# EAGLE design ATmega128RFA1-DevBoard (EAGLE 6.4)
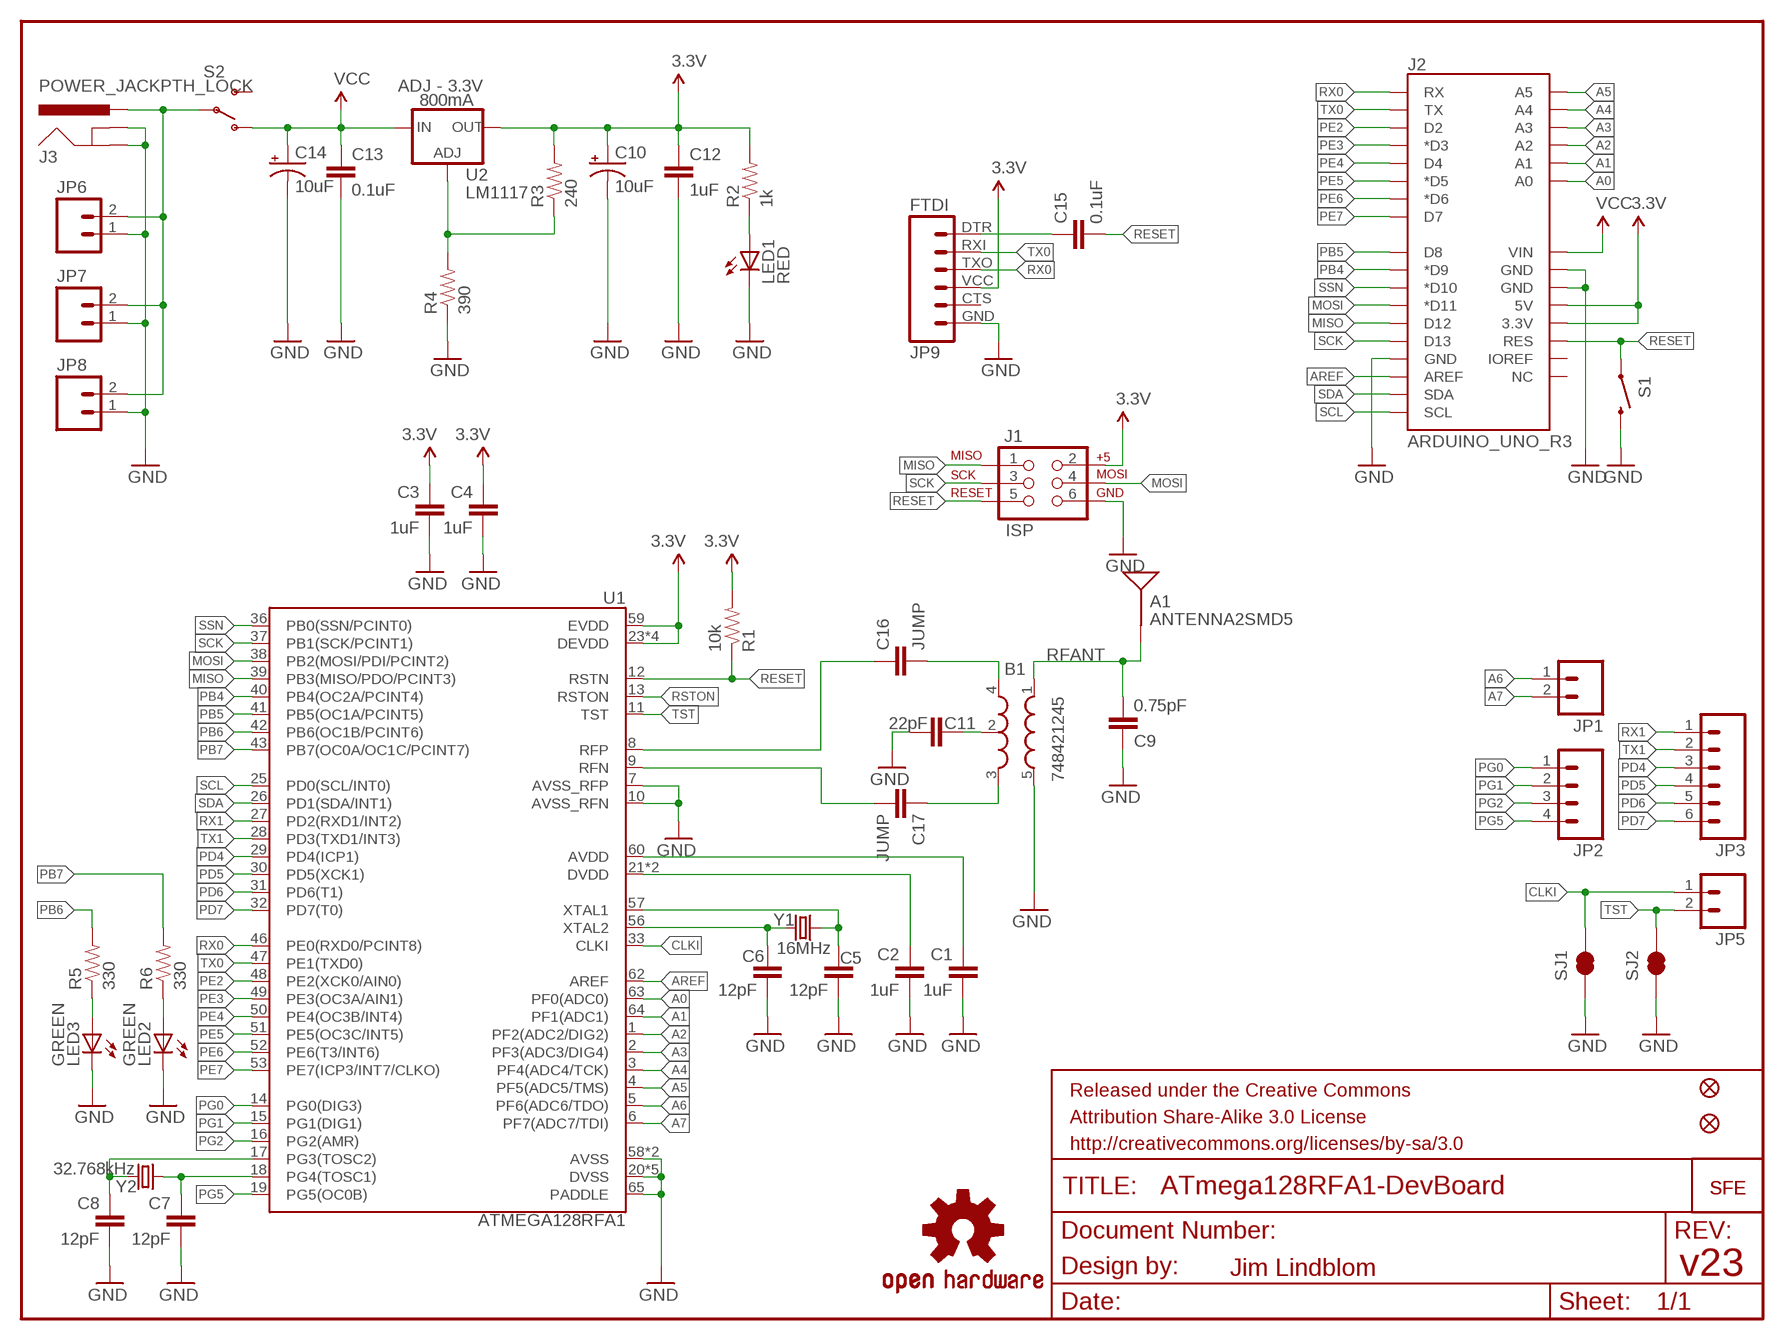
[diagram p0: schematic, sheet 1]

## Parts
A1  ANTENNA2SMD5  [ANTENNA-CHIP5]
B1  748421245  BALUN0805  [BALUN]
C1  1uF  CAP0402-CAP  [0402-CAP]
C2  1uF  CAP0402-CAP  [0402-CAP]
C3  1uF  CAP0402-CAP  [0402-CAP]
C4  1uF  CAP0402-CAP  [0402-CAP]
C5  12pF  CAP0402-CAP  [0402-CAP]
C6  12pF  CAP0402-CAP  [0402-CAP]
C7  12pF  CAP0402-CAP  [0402-CAP]
C8  12pF  CAP0402-CAP  [0402-CAP]
C9  0.75pF  CAP0402-CAP  [0402-CAP]
C10  10uF  CAP_POL1206  [EIA3216]
C11  22pF  CAP0402-CAP  [0402-CAP]
C12  1uF  CAP0402-CAP  [0402-CAP]
C13  0.1uF  CAP0402-CAP  [0402-CAP]
C14  10uF  CAP_POL1206  [EIA3216]
C15  0.1uF  CAP0402-CAP  [0402-CAP]
C16  JUMP  CAP0402-CAP  [0402-CAP]
C17  JUMP  CAP0402-CAP  [0402-CAP]
FID1  FIDUCIALUFIDUCIAL  [MICRO-FIDUCIAL]
FID2  FIDUCIALUFIDUCIAL  [MICRO-FIDUCIAL]
J1  ISP  AVR_SPI_PRG_6NS  [2X3-NS]
J2  ARDUINO_UNO_R3  [ARDUINO_UNO_R3]
J3  POWER_JACKPTH_LOCK  [POWER_JACK_PTH_LOCK]
JP1  M021X02_NO_SILK  [1X02_NO_SILK]
JP2  M041X04_NO_SILK  [1X04_NO_SILK]
JP3  M06SIP-NS  [1X06_NS]
JP4  LOGO-SFENEW  [SFE-NEW-WEBLOGO]
JP5  M021X02_NO_SILK  [1X02_NO_SILK]
JP6  M02JST-PTH-2  [JST-2-PTH]
JP7  M021X02_NO_SILK  [1X02_NO_SILK]
JP8  M023.5MM-NO_SILK  [SCREWTERMINAL-3.5MM-2-NS]
JP9  FTDI  FTDI_BASICPTH  [FTDI_BASIC]
JP10  LOGO-SFENEW  [SFE-NEW-WEBLOGO]
LED1  RED  LED0603  [LED-0603]
LED2  GREEN  LED0603  [LED-0603]
LED3  GREEN  LED0603  [LED-0603]
R1  10k  RESISTOR0402-RES  [0402-RES]
R2  1k  RESISTOR0402-RES  [0402-RES]
R3  240  RESISTOR0402-RES  [0402-RES]
R4  390  RESISTOR0402-RES  [0402-RES]
R5  330  RESISTOR0402-RES  [0402-RES]
R6  330  RESISTOR0402-RES  [0402-RES]
S1  SWITCH-MOMENTARY-2SMD  [TACTILE_SWITCH_SMD]
S2  SWITCH-SPST-SMD-A  [SWITCH-SPST-SMD-A]
SJ1  SOLDERJUMPERTRACE  [SJ_2S-TRACE]
SJ2  SOLDERJUMPERTRACE  [SJ_2S-TRACE]
U1  ATMEGA128RFA1  [QFN-64]
U2  LM1117  V_REG_317SMD  [SOT223]
U$1  OSHW-LOGOS  [OSHW-LOGO-S]
Y1  16MHz  CRYSTAL5X3  [CRYSTAL-SMD-5X3]
Y2  32.768kHz  CRYSTAL32-SMD  [CRYSTAL-32KHZ-SMD]

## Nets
3.3V: C3.1 C4.1 C10.A(+) C12.1 J1.2 J2.3.3V J2.5V JP9.VCC R1.2 R2.2 R3.2 U1.23(DEVDD) U1.34(DEVDD) U1.44(DEVDD) U1.54(DEVDD) U1.59(EVDD) U2.2(OUT)
A0: J2.A0 U1.63(PF0(ADC0))
A1: J2.A1 U1.64(PF1(ADC1))
A2: J2.A2 U1.1(PF2(ADC2/DIG2))
A3: J2.A3 U1.2(PF3(ADC3/DIG4))
A4: J2.A4 U1.3(PF4(ADC4/TCK))
A5: J2.A5 U1.4(PF5(ADC5/TMS))
A6: JP1.1 U1.5(PF6(ADC6/TDO))
A7: JP1.2 U1.6(PF7(ADC7/TDI))
AREF: J2.AREF U1.62(AREF)
AVDD: C1.1 U1.60(AVDD)
CLKI: JP5.1 SJ1.2 U1.33(CLKI)
DTR: C15.1 JP9.DTR
DVDD: C2.1 U1.21(DVDD) U1.22(DVDD)
FB: R3.1 R4.2 U2.1(ADJ)
GND: B1.5(GND) C1.2 C2.2 C3.2 C4.2 C5.2 C6.2 C7.2 C8.2 C9.1 C10.C(-) C11.2 C12.2 C13.2 C14.C(-) J1.6 J2.GND@0(GND) J2.GND@1(GND) J2.GND@2(GND) J3.GND J3.GNDBREAK JP6.1 JP7.1 JP8.1 JP9.GND LED1.C LED2.C LED3.C R4.1 S1.3 SJ1.1 SJ2.1 U1.7(AVSS_RFP) U1.10(AVSS_RFN) U1.20(DVSS) U1.24(DVSS) U1.35(DVSS) U1.45(DVSS) U1.55(DVSS) U1.58(AVSS) U1.61(AVSS) U1.65(PADDLE)
MISO: J1.1 J2.D12 U1.39(PB3(MISO/PDO/PCINT3))
MOSI: J1.4 J2.D11(*D11) U1.38(PB2(MOSI/PDI/PCINT2))
N$2: LED1.A R2.1
N$3: C5.1 U1.57(XTAL1) Y1.3
N$4: C6.1 U1.56(XTAL2) Y1.1
N$5: C7.1 U1.18(PG4(TOSC1)) Y2.X1
N$6: C8.1 U1.17(PG3(TOSC2)) Y2.X2
N$7: B1.2(GND) C11.1
N$8: LED3.A R5.1
N$9: J3.PWR JP6.2 JP7.2 JP8.2 S2.2(P)
N$10: B1.4(OUT1) C16.2
N$11: B1.3(OUT2) C17.1
N$13: LED2.A R6.1
PB4: J2.D9(*D9) U1.40(PB4(OC2A/PCINT4))
PB5: J2.D8 U1.41(PB5(OC1A/PCINT5))
PB6: R5.2 U1.42(PB6(OC1B/PCINT6))
PB7: R6.2 U1.43(PB7(OC0A/OC1C/PCINT7))
PD4: JP3.3 U1.29(PD4(ICP1))
PD5: JP3.4 U1.30(PD5(XCK1))
PD6: JP3.5 U1.31(PD6(T1))
PD7: JP3.6 U1.32(PD7(T0))
PE2: J2.D2 U1.48(PE2(XCK0/AIN0))
PE3: J2.D3(*D3) U1.49(PE3(OC3A/AIN1))
PE4: J2.D4 U1.50(PE4(OC3B/INT4))
PE5: J2.D5(*D5) U1.51(PE5(OC3C/INT5))
PE6: J2.D6(*D6) U1.52(PE6(T3/INT6))
PE7: J2.D7 U1.53(PE7(ICP3/INT7/CLKO))
PG0: JP2.1 U1.14(PG0(DIG3))
PG1: JP2.2 U1.15(PG1(DIG1))
PG2: JP2.3 U1.16(PG2(AMR))
PG5: JP2.4 U1.19(PG5(OC0B))
RESET: C15.2 J1.5 J2.RES R1.1 S1.1 U1.12(RSTN)
RFANT: A1.FEED(SIGNAL) B1.1(IN) C9.2
RFN: C17.2 U1.9(RFN)
RFP: C16.1 U1.8(RFP)
RSTON: U1.13(RSTON)
RX0: J2.RX JP9.TXO U1.46(PE0(RXD0/PCINT8))
RX1: JP3.1 U1.27(PD2(RXD1/INT2))
SCK: J1.3 J2.D13 U1.37(PB1(SCK/PCINT1))
SCL: J2.SCL U1.25(PD0(SCL/INT0))
SDA: J2.SDA U1.26(PD1(SDA/INT1))
SSN: J2.D10(*D10) U1.36(PB0(SSN/PCINT0))
TST: JP5.2 SJ2.2 U1.11(TST)
TX0: J2.TX JP9.RXI U1.47(PE1(TXD0))
TX1: JP3.2 U1.28(PD3(TXD1/INT3))
VCC: C13.1 C14.A(+) J2.VIN S2.1(O) U2.3(IN)
Unconnected: J2.IOREF J2.NC JP9.CTS S2.3(S)

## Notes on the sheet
- ADJ - 3.3V
- 800mA
- Jim Lindblom | v23

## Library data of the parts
A1 = SparkFun-RF:ANTENNA2: Chip antenna
B1 = SparkFun-RF:BALUN: 0805 footprint balun- Ember 351/357
C1-C9 C11-C13 C15 = SparkFun-Passives:CAP: Capacitor
C10 C14 = SparkFun-Passives:CAP_POL: Capacitor Polarized
C16 C17 = SparkFun:CAP: Capacitor
FID1 FID2 = SparkFun-Aesthetics:FIDUCIAL: Fiducial Alignment Points
J1 = SparkFun-Connectors:AVR_SPI_PRG_6: AVR ISP 6 Pin This is the reduced ISP connector for AVR programming. Common on Arduino. This footprint will take up less PCB space and can be used with a 10-pin to 6-pin adapter such as SKU: BOB-08508
J2 = SparkFun-Boards:ARDUINO_UNO_R3: Arduino Uno R3 This includes the two extra pins on the 8-AREF header (SDA and SCL), as well as the 2 extra pins on the power header (IOREF and NC).
J3 = SparkFun-Connectors:POWER_JACK: Power Jack This is the standard 5.5mm barrel jack for power. The PTH is the most common, proven, reliable, footprint. The Slot footprint only works if the mill layer is transmitted to the PCB fab house so be warned. Spark Fun Electronics SKU : PRT-00119 SMT: CONN-08106 Mating wall wart : TOL-00298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
JP1 JP5-JP8 = SparkFun-Connectors:M02: Header 2
JP2 = SparkFun-Connectors:M04: Header 4 Standard 4-pin 0.1" header. Use with straight break away headers (SKU : PRT-00116), right angle break away headers (PRT-00553), swiss pins (PRT-00743), machine pins (PRT-00117), and female headers (PRT-00115). Molex polarized connector foot print use with SKU : PRT-08231 with associated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
JP3 = SparkFun-Connectors:M06: Header 6 Standard 6-pin 0.1" header. Use with straight break away headers (SKU : PRT-00116), right angle break away headers (PRT-00553), swiss pins (PRT-00743), machine pins (PRT-00117), and female headers (PRT-00115). Molex polarized connector foot print use with SKU : PRT-08094 with associated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
JP4 JP10 = SparkFun-Aesthetics:LOGO-SFE: Spark Fun Electronics PCB Logo
JP9 = SparkFun-Connectors:FTDI_BASIC: FTDI Basic header with labels
LED1-LED3 = SparkFun-LED:LED: LEDs
R1 R2 = SparkFun-Passives:RESISTOR: Resistor
R3-R6 = SparkFun:RESISTOR: Resistor
S1 = SparkFun-Electromechanical:SWITCH-MOMENTARY-2: Various NO switches- pushbuttons, reed, etc
S2 = SparkFun:SWITCH-SPST: SPST Switch Simple slide switch. Spark Fun Electronics SKU : COM-00102
SJ1 SJ2 = SparkFun-Passives:SOLDERJUMPER: Solder Jumper
U1 = SparkFun-DigitalIC:ATMEGA128RFA1: ATmega128RFA1 8-bit AVR Microcontroller with Low Power 2.4GHz Transceiver for ZigBee and IEEE 802.15.4
U2 = SparkFun:V_REG_317: Voltage Regulator Standard LM317 adjustable voltage regulator. AOI (Adjust Output Input). Google 'LM317 Calculator' for easy to use app to get the two resistor values needed. 240/720 for 5V output. 240/390 for 3.3V output. Spark Fun Electronics SKU : COM-00527
U$1 = SparkFun-Aesthetics:OSHW-LOGO: Open Source Hardware Logo This logo indicates the piece of hardware it is found on incorporates a OSHW license and/or adheres to the definition of open source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
Y1 Y2 = SparkFun-FreqCtrl:CRYSTAL: Various standard crystals. Proven footprints. Spark Fun Electronics SKU : COM-00534

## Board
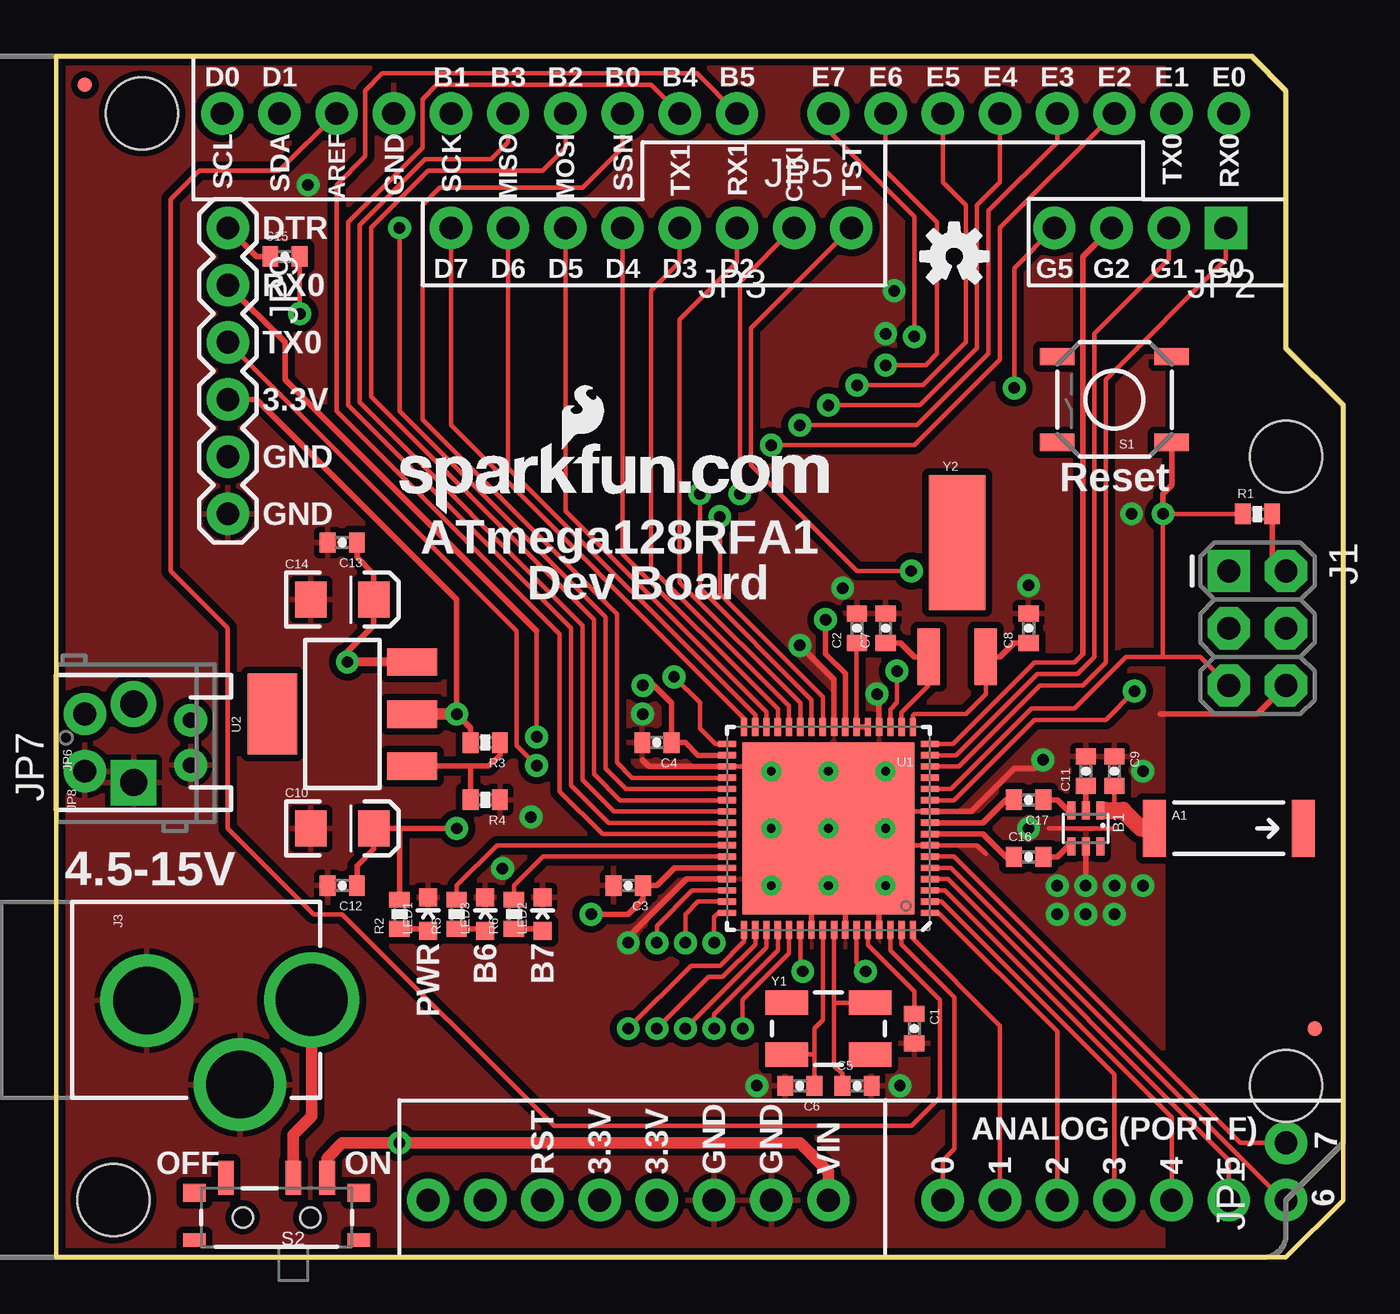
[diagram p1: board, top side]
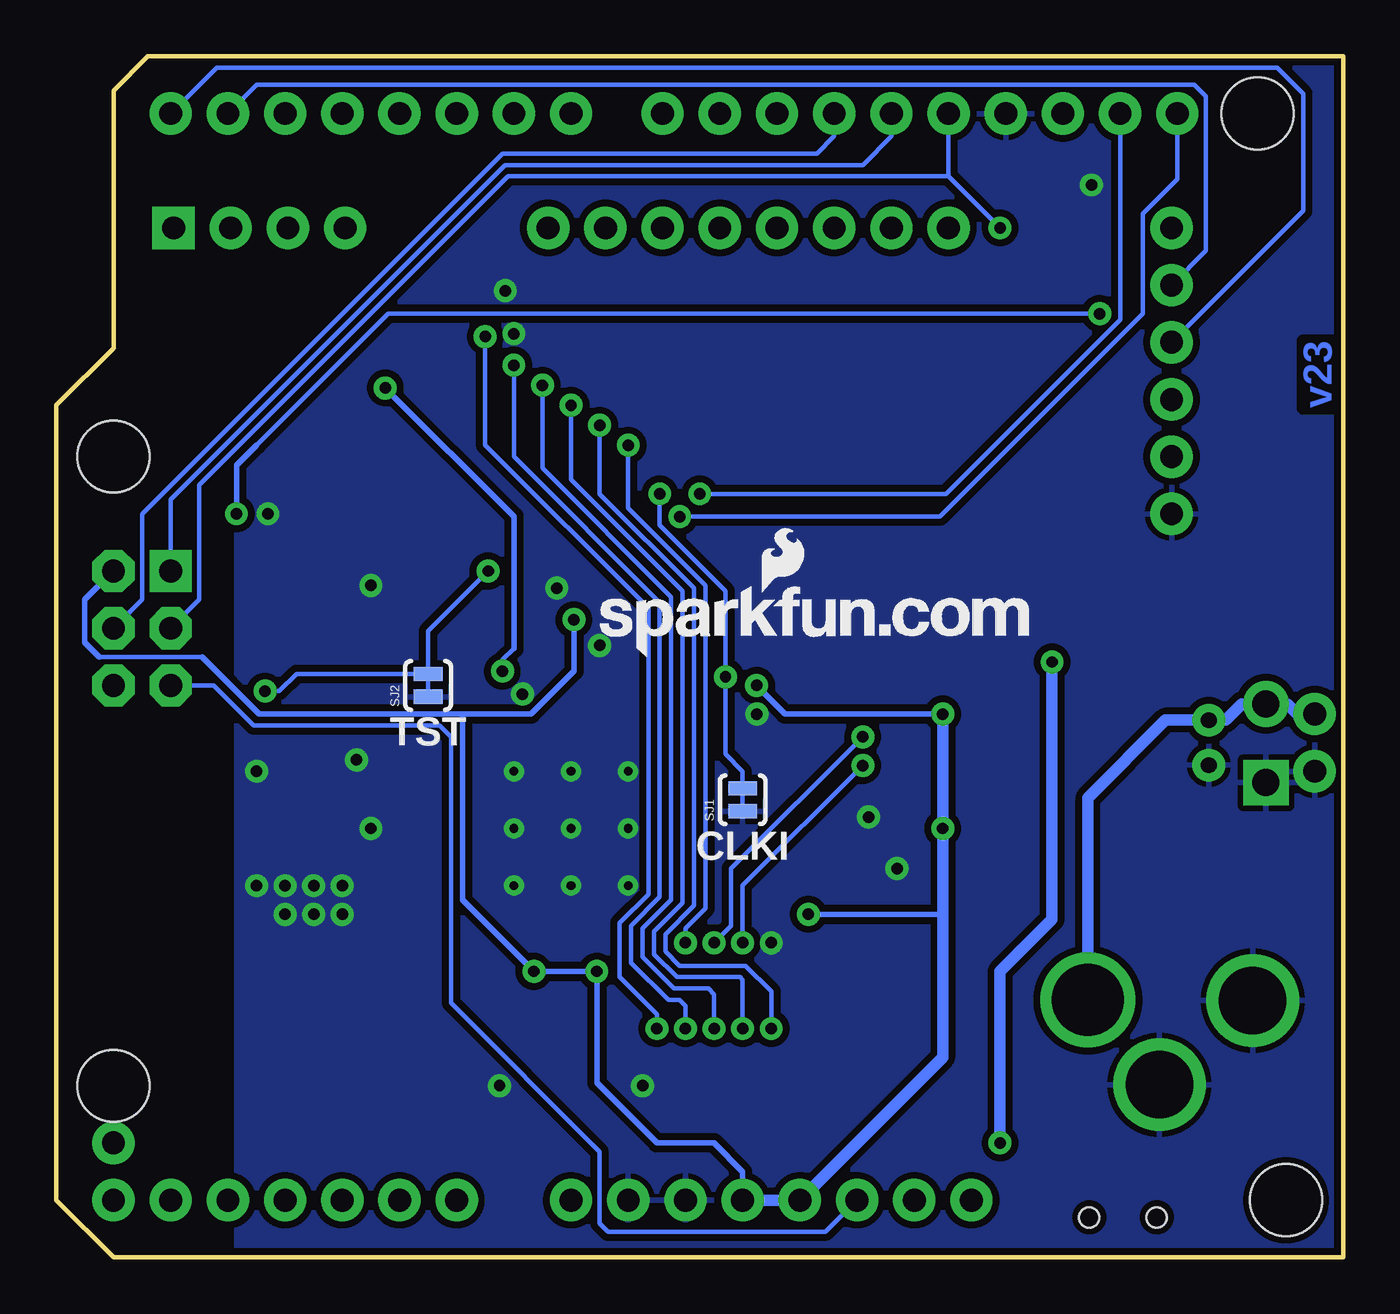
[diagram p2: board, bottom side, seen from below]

Size 57.15 x 53.34 mm. Coordinates in mm from the lower left corner, seen from the top.
Outline: 0,53.34 0,0 54.61,0 57.15,2.54 57.15,37.85 54.61,40.39 54.61,51.82 53.09,53.34 0,53.34
Copper layers (1*16): Top 0.035mm / dielectric 1.5mm / Bottom 0.035mm
Design rules "SparkFun": minimum track width 7mil, minimum drill 15mil, track to track 8mil, track to pad 8mil, pad to pad 8mil, via to via 8mil, smd to smd 8mil, copper to edge 8mil, drill to drill 8mil, minimum pad ring 12mil, minimum via ring 10mil, stop-mask expansion 4mil, vias tented up to drill 20mil, thermal gap 10mil

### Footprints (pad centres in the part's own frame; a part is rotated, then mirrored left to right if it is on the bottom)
ANTENNA-CHIP5 = smd 1.016 x 2.54: FEED -3.302,0; NC 3.302,0
BALUN = smd 0.35 x 0.8: 1 -0.65,-0.8; 2 0,-0.8; 3 0.65,-0.8; 4 0.65,0.8; 5 0,0.8; 6 -0.65,0.8
0402-CAP = smd 0.7 x 0.9: 1 -0.65,0; 2 0.65,0
EIA3216 = smd 1.4 x 1.6: A 1.4,0; C -1.4,0
MICRO-FIDUCIAL = smd 0.635 x 0.635: 1 0,0
2X3-NS = drill 1.016 pad 1.88 square: 1 -2.54,-1.27 | drill 1.016 pad 1.88 octagon: 2 -2.54,1.27; 3 0,-1.27; 4 0,1.27; 5 2.54,-1.27; 6 2.54,1.27
ARDUINO_UNO_R3 = drill 1.016 pad 1.88: 3.3V 35.56,2.54; 5V 38.1,2.54; A0 50.8,2.54; A1 53.34,2.54; A2 55.88,2.54; A3 58.42,2.54; A4 60.96,2.54; A5 63.5,2.54; AREF 23.876,50.8; D2 58.42,50.8; D3 55.88,50.8; D4 53.34,50.8; D5 50.8,50.8; D6 48.26,50.8; D7 45.72,50.8; D8 41.656,50.8; D9 39.116,50.8; D10 36.576,50.8; D11 34.036,50.8; D12 31.496,50.8; D13 28.956,50.8; GND@0 40.64,2.54; GND@1 43.18,2.54; GND@2 26.416,50.8; IOREF 30.48,2.54; NC 27.94,2.54; RES 33.02,2.54; RX 63.5,50.8; SCL 18.796,50.8; SDA 21.336,50.8; TX 60.96,50.8; VIN 45.72,2.54 | hole 3.2: 15.24,50.8; 13.97,2.54; 66.04,7.62; 66.04,35.56
POWER_JACK_PTH_LOCK = drill 2.997 pad 4.115: GND 0.025,6.557; GNDBREAK 3.762,10.7 | drill 3.2 pad 4.115: PWR 0,13.878
1X02_NO_SILK = drill 1.016 pad 1.88: 1 0,0; 2 2.54,0
1X04_NO_SILK = drill 1.016 pad 1.88 square: 1 0,0 | drill 1.016 pad 1.88: 2 2.54,0; 3 5.08,0; 4 7.62,0
1X06_NS = drill 1.016 pad 1.88: 1 0,0; 2 2.54,0; 3 5.08,0; 4 7.62,0; 5 10.16,0; 6 12.7,0
JST-2-PTH = drill 0.7 pad 1.448: 1 -1,0; 2 1,0
SCREWTERMINAL-3.5MM-2-NS = drill 1.2 pad 2.032 square: 1 0,0 | drill 1.2 pad 2.032: 2 3.5,0
FTDI_BASIC = drill 1.016 pad 1.88: CTS 10.16,0; DTR 0,0; GND 12.7,0; RXI 2.54,0; TXO 5.08,0; VCC 7.62,0
LED-0603 = smd 0.8 x 0.8: A 0,-0.75; C 0,0.75
0402-RES = smd 0.7 x 0.9: 1 -0.65,0; 2 0.65,0
TACTILE_SWITCH_SMD = smd 1.524 x 0.762: 1 -2.54,1.905; 2 2.54,1.905; 3 -2.54,-1.905; 4 2.54,-1.905
SWITCH-SPST-SMD-A = smd 0.7 x 1.5: 1 -2.25,-1.75; 2 -0.75,-1.75; 3 2.25,-1.75 | smd 1 x 0.6: GND1 -3.65,1; GND3 3.65,1 | smd 1 x 0.8: GND2 -3.65,-1.1; GND4 3.65,-1.1 | hole 0.9: -1.5,0; 1.5,0
SJ_2S-TRACE = smd 0.635 x 1.27: 1 -0.508,0; 2 0.508,0
QFN-64 = smd 0.8 x 0.28: 1 -4.5,3.75; 2 -4.5,3.25; 3 -4.5,2.75; 4 -4.5,2.25; 5 -4.5,1.75; 6 -4.5,1.25; 7 -4.5,0.75; 8 -4.5,0.25; 9 -4.5,-0.25; 10 -4.5,-0.75; 11 -4.5,-1.25; 12 -4.5,-1.75; 13 -4.5,-2.25; 14 -4.5,-2.75; 15 -4.5,-3.25; 16 -4.5,-3.75; 33 4.5,-3.75; 34 4.5,-3.25; 35 4.5,-2.75; 36 4.5,-2.25; 37 4.5,-1.75; 38 4.5,-1.25; 39 4.5,-0.75; 40 4.5,-0.25; 41 4.5,0.25; 42 4.5,0.75; 43 4.5,1.25; 44 4.5,1.75; 45 4.5,2.25; 46 4.5,2.75; 47 4.5,3.25; 48 4.5,3.75 | smd 0.28 x 0.8: 17 -3.75,-4.5; 18 -3.25,-4.5; 19 -2.75,-4.5; 20 -2.25,-4.5; 21 -1.75,-4.5; 22 -1.25,-4.5; 23 -0.75,-4.5; 24 -0.25,-4.5; 25 0.25,-4.5; 26 0.75,-4.5; 27 1.25,-4.5; 28 1.75,-4.5; 29 2.25,-4.5; 30 2.75,-4.5; 31 3.25,-4.5; 32 3.75,-4.5; 49 3.75,4.5; 50 3.25,4.5; 51 2.75,4.5; 52 2.25,4.5; 53 1.75,4.5; 54 1.25,4.5; 55 0.75,4.5; 56 0.25,4.5; 57 -0.25,4.5; 58 -0.75,4.5; 59 -1.25,4.5; 60 -1.75,4.5; 61 -2.25,4.5; 62 -2.75,4.5; 63 -3.25,4.5; 64 -3.75,4.5 | smd 7.65 x 7.65: 65 0,0
SOT223 = smd 1.219 x 2.235: 1 -2.311,-3.099; 2 0,-3.099; 3 2.311,-3.099 | smd 3.6 x 2.2: 4 0,3.099
CRYSTAL-SMD-5X3 = smd 1.9 x 1.1: 1 -1.85,-1.15; 2 1.85,-1.15; 3 1.85,1.15; 4 -1.85,1.15
CRYSTAL-32KHZ-SMD = smd 2.5 x 6: SHEILD 0,5.08 | smd 1 x 2.5: X1 -1.27,0; X2 1.27,0

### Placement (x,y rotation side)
A1  52.07,19.05 0 top
B1  45.72,19.05 180 top
C1  38.1,10.16 270 top
C2  35.56,27.94 90 top
C3  25.4,16.51 180 top
C4  26.67,22.86 180 top
C5  35.56,7.62 0 top
C6  33.02,7.62 180 top
C7  36.83,27.94 90 top
C8  43.18,27.94 90 top
C9  46.99,21.59 270 top
C10  12.7,19.05 0 top
C11  45.72,21.59 90 top
C12  12.7,16.51 180 top
C13  12.7,31.75 180 top
C14  12.7,29.21 0 top
C15  10.16,44.45 0 top
C16  43.18,17.78 0 top
C17  43.18,20.32 180 top
FID1  1.27,52.07 0 top
FID2  55.88,10.16 0 top
J1  53.34,27.94 270 top
J2  -11.43,0 0 top
J3  -2.54,11.43 270 top
JP1  54.61,2.54 90 top
JP2  51.94,45.72 180 top
JP3  30.23,45.72 180 top
JP4  33.02,26.67 0 bottom
JP5  32.77,45.72 0 top
JP6  5.97,22.86 90 top
JP7  1.27,21.59 90 top
JP8  3.43,21.08 90 top
JP9  7.62,45.72 270 top
JP10  15.24,33.02 0 top
LED1  16.51,15.24 0 top
LED2  21.59,15.24 0 top
LED3  19.05,15.24 0 top
R1  53.34,33.02 0 top
R2  15.24,15.24 90 top
R3  19.05,22.86 180 top
R4  19.05,20.32 180 top
R5  17.78,15.24 90 top
R6  20.32,15.24 90 top
S1  46.99,38.1 180 top
S2  9.78,1.78 180 top
SJ1  26.67,20.32 90 bottom
SJ2  40.64,25.4 90 bottom
U1  34.29,19.05 180 top
U2  12.7,24.13 90 top
U$1  39.88,44.45 0 top
Y1  34.29,10.16 0 top
Y2  40.01,26.67 0 top

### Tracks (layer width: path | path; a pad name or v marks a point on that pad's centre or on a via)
3.3V  (via drill 0.51)
  Top 0.203: U1.54 33.04,12.81 v33.15,12.7 | U1.59 35.54,13.1 v35.94,12.7
  Top 0.254: U1.34 28.5,22.3 27.94,22.86 C4.1 27.32,24.62 26.54,25.4 v26.05,25.4 | U1.44 27.46,17.3 26.67,16.51 C3.1 26.05,15.89 25.4,15.24 v23.75,15.24 | 15.24,19.05 C10.A 14.1,18.13 13.35,17.38 C12.1 | 15.24,19.05 v17.78,19.05 | R1.2 53.99,31.1 J1.2 | R2.2 15.24,19.05 | JP9.VCC 8.89,38.1 17.78,29.21 v17.78,24.13 18.4,23.51 R3.2 | U1.23 35.04,25.92 34.16,26.8 v34.16,28.32
  Top 0.508: U2.2 v17.78,24.13
  Bottom 0.203: 50.67,26.67 55.24,26.67
  Bottom 0.254: v23.75,15.24 17.78,15.24 | 39.12,24.13 39.12,15.88 v35.94,12.7 v33.15,12.7 33.15,7.75 30.48,5.08 27.94,5.08 26.67,3.81 J2.5V | 39.12,24.13 36.07,24.13 34.16,26.04 v34.16,28.32 | 39.12,24.13 48.13,24.13 50.67,26.67 | 55.24,26.67 55.88,27.3 55.88,29.21 J1.2 | v17.78,24.13 24.78,24.13 v26.05,25.4
  Bottom 0.508: v17.78,24.13 v17.78,19.05 17.78,15.24 17.78,8.89 J2.3.3V J2.5V
A0
  Top 0.203: J2.A0 39.37,4.32 39.88,4.83 39.88,11.56 37.54,13.89 U1.63
A1
  Top 0.203: J2.A1 41.91,10.29 38.04,14.16 U1.64
A2
  Top 0.203: U1.1 39.18,15.3 44.45,10.03 J2.A2
A3
  Top 0.203: U1.2 39.32,15.8 46.99,8.13 J2.A3
A4
  Top 0.203: U1.3 39.45,16.3 49.53,6.22 J2.A4
A5
  Top 0.203: U1.4 39.59,16.8 52.07,4.32 J2.A5
A6
  Top 0.203: U1.5 39.72,17.3 54.48,2.54 JP1.1
A7
  Top 0.203: U1.6 39.86,17.8 52.58,5.08 JP1.2
AREF
  Top 0.203: J2.AREF 9.91,48.26 6.35,48.26 5.08,46.99 5.08,30.48 7.62,27.94 7.62,19.05 11.43,15.24 12.7,15.24 22.1,5.84 37.97,5.84 39.24,7.11 39.24,11.43 37.04,13.63 U1.62
AVDD
  Top 0.203: U1.60 36.04,13.87 38.1,11.81 C1.1
CLKI  (via drill 0.51)
  Top 0.203: v30.35,33.91 30.35,43.31 JP5.1 | U1.33 29.27,22.8 28.57,23.5 28.57,24.64 v27.43,25.78
  Bottom 0.203: SJ1.2 26.67,21.59 27.43,22.35 v27.43,25.78 27.43,29.59 30.35,32.51 v30.35,33.91
DTR
  Top 0.254: C15.1 8.89,44.45 JP9.DTR
DVDD
  Top 0.203: U1.22 35.54,27.16
  Top 0.254: U1.21 U1.22 | 35.54,27.16 35.56,27.18 C2.1
FB
  Top 0.254: R3.1 19.7,22.32 19.2,21.82 18.4,21.82 | R4.2 18.4,21.82 | 18.4,21.82 U2.1
GND  (via drill 0.38, 0.51)
  Top 0.203: 35.97,19.05 v36.83,19.05 37.58,18.3 U1.7 40.88,18.3 41.27,17.91 | v36.83,21.59 v34.29,21.59 v31.75,21.59 31.54,21.8 U1.35 | 36.32,15.49 36.32,16 v36.83,16.51 36.54,16.22 36.54,15.46 | 35.04,15.48 35.04,15.76 v34.29,16.51 | U1.10 37.58,19.8 | 46.86,19.05 44.07,19.05
  Top 0.254: 39.26,19.8 39.24,19.81 | U1.10 39.37,19.8 | 39.37,19.8 40.63,19.8 42.55,21.72 43.43,21.72 v43.81,22.1 | U1.61 36.54,15.46 | U1.58 35.04,15.48 | U1.55 33.54,15.48 34.29,16.23 v34.29,16.51 v31.75,16.51 | U1.24 34.54,25.66 v33.02,27.18 | U1.35 26.33,21.8 26.04,22.1 | U1.45 27.98,16.8 25.65,14.48 | 37.58,19.8 v36.83,19.05 | 38.86,19.81 39.24,19.81 | 39.36,19.81 40.13,19.81 | B1.5 v45.72,16.51 | J1.6 53.34,24.13 49.02,24.13 | U1.20 36.54,24.93 v36.45,25.02 | 39.24,19.81 39.36,19.81 | 39.36,19.81 39.37,19.8
  other vias: 34.29,19.05 31.75,19.05 25.4,13.97 44.45,16.51 43.18,19.05 19.81,17.27 11.18,47.62 26.04,24.13 37.47,7.62 31.11,7.62 44.45,15.24 46.99,16.51 46.99,15.24 45.72,15.24 21.08,19.56 47.75,33.02 43.18,29.84 34.92,29.72 36.83,41.02 48.26,21.59 48.26,16.51 37.21,42.93
  pour Top (isolate 0.305, rank 2): 0,53.34 0,0 49.15,0 49.15,53.34
  pour Bottom (isolate 0.305): 0,53.34 49.15,53.34 49.15,0 0,0
MISO
  Top 0.203: U1.39 24.78,19.8 23.37,21.21 23.37,28.07 13.46,37.97 13.46,45.85 16.38,48.77 19.3,48.77 20.07,49.53 J2.D12
  Bottom 0.203: J1.1 52.07,33.66 37.21,48.51 21.34,48.51 20.07,49.78 J2.D12
MOSI
  Top 0.203: U1.38 25.04,20.3 23.88,21.46 23.88,28.32 13.97,38.23 13.97,45.72 16.51,48.26 21.59,48.26 22.61,49.28 J2.D11
  Bottom 0.203: J1.4 53.34,29.21 53.34,33.02 37.34,49.02 23.37,49.02 22.61,49.78 J2.D11
N$2
  Top 0.254: R2.1 16.41,14.59 LED1.A
N$3
  Top 0.203: C5.1 34.91,8.14 34.54,8.51 34.54,11.3 | U1.57 34.54,11.3 | 35.81,11.3 34.54,11.3
  Top 0.254: Y1.3 35.82,11.31 35.81,11.3
N$4
  Top 0.203: U1.56 34.04,10.54 33.67,10.18 33.67,9.02 | C6.1 33.67,9.02 | Y1.1 33.66,9.01 33.67,9.02
N$5
  Top 0.203: U1.18 37.54,24.2 38.73,25.4 Y2.X1
  Top 0.254: C7.1 37.48,27.29 38.1,26.67 Y2.X1
N$6
  Top 0.203: U1.17 38.04,24.07 38.1,24.13 40.39,24.13 41.27,25.02 Y2.X2
  Top 0.254: C8.1 42.53,27.29 41.91,26.67 Y2.X2
N$7
  Top 0.254: B1.2 C11.1
N$8
  Top 0.254: R5.1 18.95,14.59 LED3.A
N$9
  Top 0.508: S2.2 10.53,5.45 11.34,6.26 J3.PWR
  Bottom 0.508: JP7.2 2.03,24.13 2.48,24.58 JP8.2 4.5,24.58 5.22,23.86 JP6.2 7.89,23.86 11.34,20.41 J3.PWR
N$10
  Top 0.254: C16.2 44.45,17.78 44.92,18.25 B1.4
N$11
  Top 0.254: C17.1 44.45,20.32 44.92,19.85 B1.3
N$13
  Top 0.254: R6.1 21.49,14.59 LED2.A
PB4
  Top 0.203: U1.40 24.52,19.3 22.86,20.95 22.86,27.94 12.95,37.85 12.95,45.97 16.26,49.28 16.26,51.44 16.89,52.07 26.42,52.07 J2.D9
PB5
  Top 0.203: U1.41 24.25,18.8 22.35,20.7 22.35,27.69 12.45,37.59 12.45,47.62 13.72,48.9 13.72,51.82 14.48,52.58 28.45,52.58 J2.D8
PB6
  Top 0.203: U1.42 19.57,18.3 17.78,16.51 R5.2
PB7
  Top 0.203: U1.43 21.61,17.8 20.32,16.51 R6.2
PD4
  Top 0.203: U1.29 32.04,24.35 25.15,31.24 JP3.3
PD5
  Top 0.203: U1.30 31.54,24.21 22.61,33.15 JP3.4
PD6
  Top 0.203: U1.31 31.04,24.08 20.07,35.05 JP3.5
PD7
  Top 0.203: U1.32 30.54,23.94 17.53,36.96 JP3.6
PE2  (via drill 0.51)
  Top 0.203: v31.75,36.07 38.1,36.07 41.91,39.88 41.91,45.72 J2.D2 | v29.21,13.97 29.21,15.11 29.4,15.3 U1.48
  Bottom 0.203: v31.75,36.07 31.75,33.27 28.32,29.84 28.32,15.49 29.21,14.61 v29.21,13.97
PE3  (via drill 0.51)
  Top 0.203: v33.02,36.96 38.23,36.96 41.4,40.13 41.4,46.48 44.45,49.53 J2.D3 | U1.49 30.54,14.03 29.46,12.95 28.19,12.95 v25.4,10.16
  Bottom 0.203: v25.4,10.16 25.4,11.81 26.54,12.95 29.46,12.95 30.1,13.59 30.1,14.35 28.83,15.62 28.83,29.72 33.02,33.91 v33.02,36.96
PE4  (via drill 0.51)
  Top 0.203: v34.29,37.85 38.35,37.85 40.89,40.39 40.89,46.74 41.91,47.75 J2.D4 | U1.50 31.04,13.89 29.59,12.45 28.96,12.45 v26.67,10.16
  Bottom 0.203: v26.67,10.16 26.67,12.32 26.8,12.45 29.59,12.45 30.61,13.46 30.61,14.48 29.34,15.75 29.34,29.59 34.29,34.54 v34.29,37.85
PE5  (via drill 0.51)
  Top 0.203: v35.56,38.73 38.48,38.73 40.39,40.64 40.39,46.74 39.37,47.75 J2.D5 | U1.51 31.54,13.76 v27.94,10.16
  Bottom 0.203: v27.94,10.16 27.94,11.68 28.19,11.94 29.72,11.94 31.11,13.34 31.11,14.61 29.84,15.88 29.84,29.34 35.56,35.05 v35.56,38.73
PE6  (via drill 0.51)
  Top 0.203: v36.83,39.62 38.61,39.62 39.12,40.13 39.12,45.97 36.83,48.26 J2.D6 | U1.52 32.04,13.62 29.21,10.79 v29.21,10.16
  Bottom 0.203: v36.83,39.62 36.83,35.56 30.35,29.08 30.35,16 31.62,14.73 31.62,13.08 29.97,11.43 29.46,11.43 29.21,11.18 v29.21,10.16
PE7  (via drill 0.51)
  Top 0.203: J2.D7 34.29,50.04 38.1,46.23 v38.1,40.89 | U1.53 32.54,13.49 30.48,11.43 v30.48,10.16
  Bottom 0.203: v38.1,40.89 38.1,36.07 30.86,28.83 30.86,16.13 32.13,14.86 32.13,12.45 30.48,10.79 v30.48,10.16
PG0
  Top 0.203: U1.14 40.09,21.8 43.69,25.4 45.59,25.4 46.61,26.42 46.61,38.99 51.94,44.32 JP2.1
PG1
  Top 0.203: U1.15 39.95,22.3 43.56,25.91 45.34,25.91 46.1,26.67 46.1,41.02 49.4,44.32 JP2.2
PG2
  Top 0.203: U1.16 39.82,22.8 43.43,26.42 45.21,26.42 45.59,26.8
  Top 0.254: 45.59,26.8 45.59,44.45 JP2.3
PG5  (via drill 0.51)
  Top 0.203: U1.19 37.04,24.34 37.34,24.64 v37.34,26.04 | v42.55,38.61 42.55,43.94 JP2.4
  Bottom 0.203: v37.34,26.04 37.34,26.54 36.83,27.05
  Bottom 0.254: 36.83,27.05 36.83,32.89 v42.55,38.61
RESET  (via drill 0.51)
  Top 0.203: U1.12 39.72,20.8 43.31,24.38 45.21,24.38 47.5,26.67 49.15,26.67 | J1.5 50.8,26.67 49.15,26.67 | R1.1 v49.15,33.02 49.15,26.67 | C15.2 v10.81,41.91
  Top 0.254: v49.15,33.02 49.15,33.91 49.53,34.29 S1.1
  Bottom 0.203: J2.RES 22.99,1.14 32.64,1.14 33.02,1.52 33.02,4.7 39.62,11.3 39.62,23.11 40.13,23.62 48.39,23.62 50.16,25.4 J1.5 | v10.81,41.91 42.42,41.91 48.26,36.07
  Bottom 0.254: 48.26,36.07 49.15,35.18 v49.15,33.02
RFANT
  Top 0.203: C9.2 46.99,19.85
  Top 0.254: B1.1 46.57,19.85
  Top 0.762: 46.57,19.85 46.99,19.85 47.37,19.85 48.17,19.05 A1.FEED
RFN
  Top 0.254: U1.9 41.14,19.3 42.16,20.32 C17.2
RFP
  Top 0.254: U1.8 41.14,18.8 42.16,17.78 C16.1
RX0  (via drill 0.51)
  Top 0.203: U1.46 28.24,16.3 26.67,14.73 v26.67,13.97 | JP9.TXO 20.45,27.81 20.45,22.73 v21.34,21.84
  Bottom 0.203: v26.67,13.97 26.67,16.51 v21.34,21.84 | J2.RX 50.04,52.83 2.92,52.83 1.78,51.69 1.78,46.48 JP9.TXO
RX1
  Top 0.203: U1.27 33.04,24.62 27.69,29.97 27.69,41.66 30.23,44.2 JP3.1
SCK  (via drill 0.51)
  Top 0.203: U1.37 25.3,20.8 24.38,21.72 24.38,28.45 15.24,37.59 v15.24,45.72
  Bottom 0.203: v15.24,45.72 17.53,48.01 | J2.D13 17.53,48.01 | J1.3 50.8,29.21 50.8,34.29 37.08,48.01 17.53,48.01
SCL  (via drill 0.51)
  Top 0.203: U1.25 34.04,24.89 29.46,29.46 v29.46,32.89
  Bottom 0.203: v29.46,32.89 17.91,32.89 8.89,41.91 8.89,46.35 7.37,47.88 J2.SCL
SDA  (via drill 0.51)
  Top 0.203: U1.26 33.54,24.75 28.57,29.72 v28.57,33.91
  Bottom 0.203: v28.57,33.91 17.65,33.91 9.91,41.66 J2.SDA
SSN
  Top 0.203: U1.36 25.56,21.3 24.89,21.97 24.89,28.57 16.26,37.21 16.26,46.74 17.02,47.5 23.37,47.5 25.15,49.28 J2.D10
TST  (via drill 0.51)
  Top 0.203: U1.11 39.86,20.3 43.43,23.88 46.61,23.88 v47.88,25.15 | JP5.2 30.86,41.27 30.86,35.18 35.56,30.48 v37.97,30.48
  Bottom 0.203: v37.97,30.48 40.64,27.81 SJ2.2 46.48,25.91 47.24,25.15 v47.88,25.15
TX0  (via drill 0.51)
  Top 0.203: U1.47 28.5,15.8 27.94,15.24 v27.94,13.97 | v21.34,23.11 21.34,27.81
  Top 0.254: 21.34,27.81 10.16,38.99 10.16,40.64 JP9.RXI
  Bottom 0.203: JP9.RXI 6.1,44.7 6.1,51.56 6.6,52.07 48.26,52.07 J2.TX | v27.94,13.97 27.18,14.73 27.18,17.27 v21.34,23.11
TX1
  Top 0.203: U1.28 32.54,24.48 26.42,30.61 26.42,42.93 27.69,44.2 JP3.2
VCC  (via drill 0.51)
  Top 0.254: v12.93,26.44 12.93,26.9 14.1,28.07 C14.A 14.1,30.36 13.35,31.11 C13.1
  Top 0.406: U2.3 v12.93,26.44
  Top 0.508: J2.VIN 34.29,3.81 33.02,5.08 v15.24,5.08 12.7,5.08 12.03,4.41 S2.1
  Bottom 0.508: v12.93,26.44 12.93,15.01 15.24,12.7 v15.24,5.08

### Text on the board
Bottom: v23
tPlace: D0 | D1 | B1 | B3 | B2 | B0 | B4 | B5 | E7 | E6 | E5 | E4 | E3 | E2 | E1 | E0 | SCL | SDA | AREF | GND | SCK | MISO | MOSI | SSN | TX0 | RX0 | TX1 | RX1 | CLKI | TST | DTR | D7 | D6 | D5 | D4 | D3 | D2 | G5 | G2 | G1 | G0 | RX0 | TX0 | 3.3V | GND | Reset | GND | ATmega128RFA1 | Dev Board | 4.5-15V | PWR | B6 | B7 | ANALOG (PORT F) | 7 | OFF | ON | RST | 3.3V | 3.3V | GND | GND | VIN | 0 | 1 | 2 | 3 | 4 | 5 | 6
bPlace: TST | CLKI

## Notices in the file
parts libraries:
SparkFun-Aesthetics: Licensing: CC v3.0 Share-Alike You are welcome to use this library for commercial purposes.
SparkFun-Aesthetics: Released under the Creative Commons
SparkFun-Aesthetics: http://creativecommons.org/licenses/by-sa/3.0
